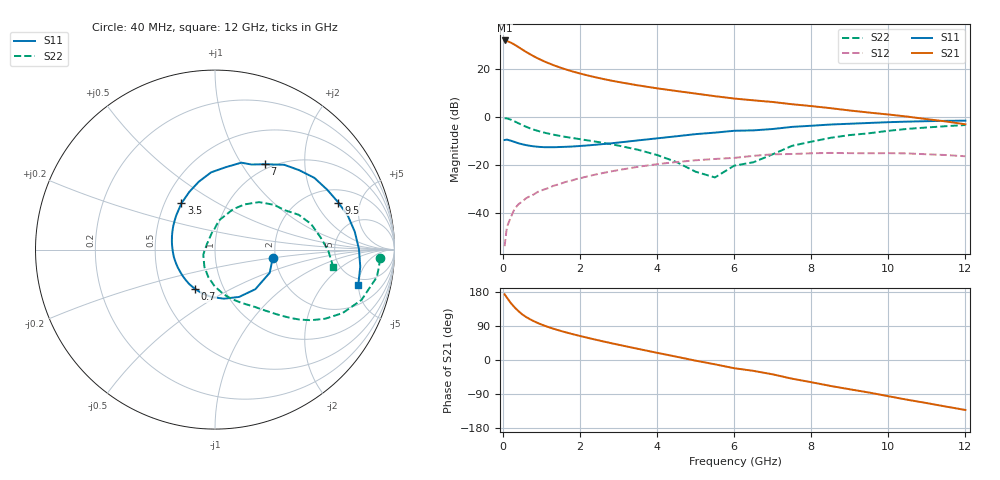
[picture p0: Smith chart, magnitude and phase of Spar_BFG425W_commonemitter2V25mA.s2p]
! Filename: 225bfg425.001
! BFG425W Field C1
! V1=8.667E-001V,V2=2.000E+000V, I1=3.585E-004A, I2=2.496E-002A
# GHz  S  MA  R 50
!  S11  S21  S12  S22
!Freq(GHz)  Mag  Ang  Mag  Ang  Mag  Ang  Mag  Ang
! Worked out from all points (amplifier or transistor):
!   44 points, 40 MHz to 12 GHz, reference 50 ohm
!   highest |S21| = 31.7 dB at 40 MHz (marker M1)
!   |S21| within 3 dB of that: start of sweep to 422.1 MHz
!   unconditionally stable (mu >= 1): 1.135 GHz to end of sweep
!   at 700 MHz: K = 0.82, MSG = 29.6 dB, |S12| = -33.2 dB
!   at 2.4 GHz: K = 1.17, MAG = 17.8 dB, |S12| = -24.2 dB
!   at 12 GHz: K = 1.34, MAG = 3.2 dB, |S12| = -16.5 dB
!   lowest NFmin = 2.10 dB at 900 GHz
!   S11 on the Smith chart (normalised r, x): 40 MHz: 1.93, -0.21; 700 MHz: 0.73, -0.34; 3.5 GHz: 0.61, +0.35; 7 GHz: 0.93, +1.27; 9.5 GHz: 2.76, +3.15; 12 GHz: 4.08, -4.95
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0.04  0.325 -8.7  38.47 173.4  0.002 71.9  0.923 -3.1
0.1  0.331 -23.0  37.46 164.5  0.005 83.3  0.915 -9.6
0.2  0.315 -44.5  34.77 150.5  0.008 75.9  0.863 -19.0
0.3  0.296 -63.0  31.36 138.8  0.012 71.6  0.794 -26.4
0.4  0.278 -79.7  27.95 128.8  0.015 68.2  0.725 -32.1
0.5  0.265 -94.3  24.86 120.2  0.017 66.0  0.664 -36.3
0.6  0.254 -106.5  22.16 113.4  0.02 64.5  0.613 -39.5
0.7  0.246 -116.8  19.89 107.5  0.022 63.4  0.569 -42.1
0.9  0.235 -134.5  16.34 97.6  0.027 61.9  0.504 -46.0
1.2  0.23 -154.2  12.75 86.1  0.033 59.9  0.438 -50.7
1.7  0.236 -178.5  9.213 71.1  0.045 56.0  0.369 -57.7
2.2  0.251 162.8  7.172 58.4  0.057 50.7  0.319 -65.7
2.8  0.277 144.2  5.628 44.6  0.072 43.4  0.266 -76.2
3.5  0.319 125.8  4.47 29.5  0.09 33.6  0.204 -90.6
4.5  0.389 103.4  3.406 8.7  0.113 18.4  0.113 -121.6
5.5  0.463 82.6  2.658 -11.4  0.131 2.5  0.054 148.7
6.5  0.516 66.7  2.179 -28.7  0.152 -10.1  0.112 92.3
7  0.551 59.7  2.011 -37.9  0.164 -17.9  0.164 82.3
8.5  0.683 35.8  1.496 -68.5  0.175 -47.0  0.361 47.2
9.5  0.736 20.9  1.212 -85.8  0.172 -63.4  0.449 29.1
10.5  0.785 7.3  0.997 -105.0  0.171 -81.8  0.554 15.0
12  0.822 -13.8  0.69 -131.9  0.149 -111.1  0.667 -8.5
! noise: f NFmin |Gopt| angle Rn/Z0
900  2.1  0.25  -166.3  0.19
2000  2.5  0.22  -152.2  0.21
